(* Logix 5000 AddOnInstructionDefinition export AKD_Drive; software revision 19.01 *)

TYPE AKD_Status :   // All connections to the drive ethernet module are established and data is successfully transferring.
STRUCT
   Profile_In_Progress : BOOL;   // Profile Move In Progress
   Block_In_Execution : BOOL;   // Block In Execution
   On_Target_Position : BOOL;   // On Target Position (1=Current Position Equals Last Target Position)
   General_Fault : BOOL;   // General Fault
   Current_Direction : BOOL;   // Current Motor Direction (0=Reverse, 1=Forward)
   Home_Level : BOOL;   // Level of Home Input
   Reg_Level : BOOL;   // Level of Registration Input
   Enable : BOOL;   // State of Enable Output
   Fault_Input_Fault : BOOL;   // Fault Input Active
   Fwd_Limit : BOOL;   // Forward Input Active
   Rev_Limit : BOOL;   // Reverse Input Active
   Positive_Limit : BOOL;   // Positive Software Limit Exceeded
   Negative_Limit : BOOL;   // Negative Software Limit Exceeded
   FE_Fault : BOOL;   // Following Error Fault
   Block_Fault : BOOL;   // Block Execution Fault
   Load_Complete : BOOL;   // Command Message Successfully Loaded
END_STRUCT
END_TYPE

TYPE AKD_Axis :   // Axis Data:
STRUCT
   Control : AKD_Control;   // Control bits to send to the drive
   Status : AKD_Status;   // Status bits received from the drive
   Input : AB:ETHERNET_MODULE_SINT_64Bytes:I:0;   // Data from the drive
   Output : AB:ETHERNET_MODULE_SINT_64Bytes:O:0;   // Data to the drive
   ResponseMsgType : SINT;   // Response type contained in latest IO response from drive. Used to check for errors
   CommandTimeout : INT;   // Time to allow for command response from drive. Dependent on scan rate and communicaiton rate
   PositionFeedback : DINT;   // Actual Position Value
   VelocityFeedback : DINT;   // Actual Velocity Value
END_STRUCT
END_TYPE

TYPE AKD_Control :   // Send Explicit Message
STRUCT
   Load_Data_Start_Profile : BOOL;   // Load Command Data / Start Profile Move
   Start_Block : BOOL;   // Execute Command block or block chain
   Incremental : BOOL;   // Incremental Position (0=Absolute, 1=Incremental)
   Direction : BOOL;   // Direction in Velocity Mode (0=Reverse, 1=Forward)
   Smooth_Stop : BOOL;   // Smooth / Controlled Stop w/ Deceleration
   Hard_Stop : BOOL;   // Hard / Immediate Stop
   Reg_Arm : BOOL;   // Arm the Registration Input
   Enable : BOOL;   // Enable Output
END_STRUCT
END_TYPE

ADD_ON_INSTRUCTION AKD_Drive   (* revision 2.0, ExecutePrescan *)
// Drive Communication
VAR_IN_OUT
   Axis_Input : AB:ETHERNET_MODULE_SINT_64Bytes:I:0; {required}
   Axis_Output : AB:ETHERNET_MODULE_SINT_64Bytes:O:0; {required}
   Axis_Internal : AKD_Axis; {required}
END_VAR
VAR
   Command_Bytes : SINT[8];
   Response_Bytes : SINT[8];
END_VAR

ROUTINE Logic   (* ladder *)
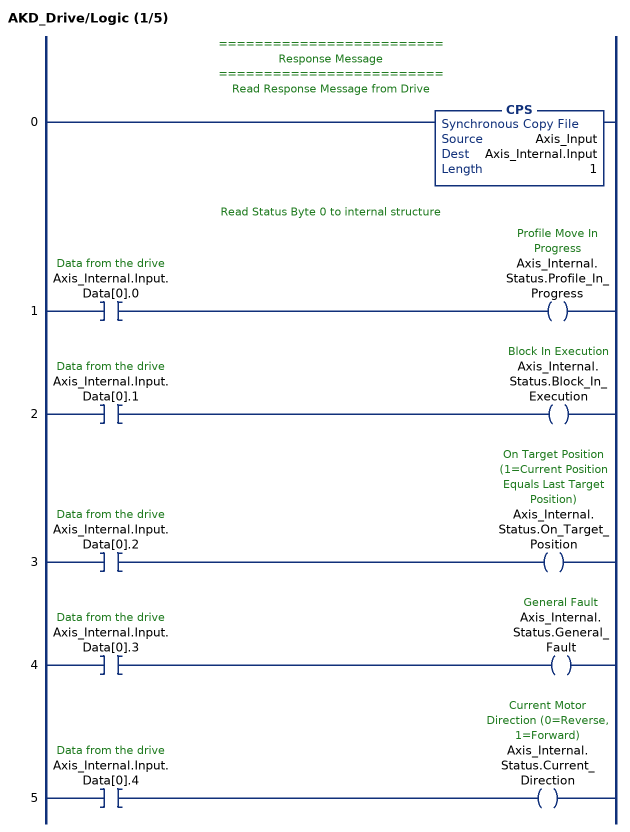
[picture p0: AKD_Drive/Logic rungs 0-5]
   // =========================
   // Response Message
   // =========================
   // Read Response Message from Drive
   0: CPS(Axis_Input,Axis_Internal.Input,1);
   // Read Status Byte 0 to internal structure
   1: XIC(Axis_Internal.Input.Data[0].0)OTE(Axis_Internal.Status.Profile_In_Progress);
   2: XIC(Axis_Internal.Input.Data[0].1)OTE(Axis_Internal.Status.Block_In_Execution);
   3: XIC(Axis_Internal.Input.Data[0].2)OTE(Axis_Internal.Status.On_Target_Position);
   4: XIC(Axis_Internal.Input.Data[0].3)OTE(Axis_Internal.Status.General_Fault);
   5: XIC(Axis_Internal.Input.Data[0].4)OTE(Axis_Internal.Status.Current_Direction);
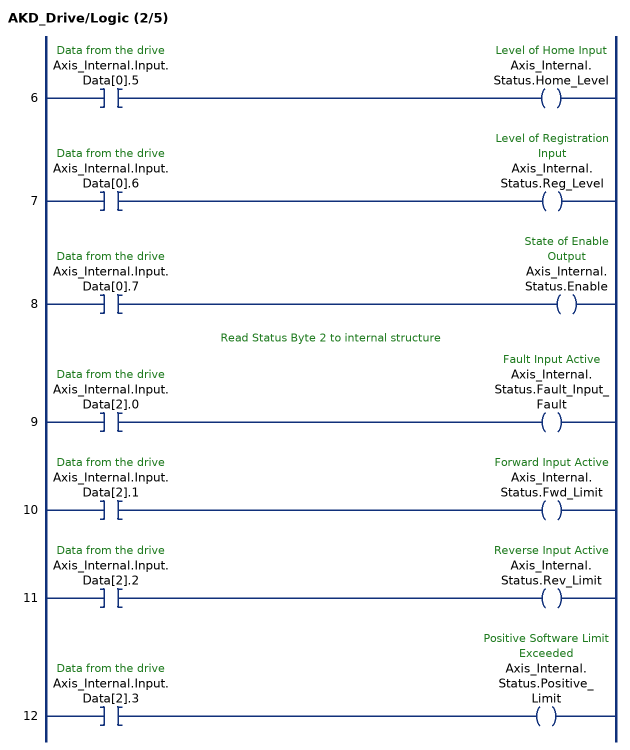
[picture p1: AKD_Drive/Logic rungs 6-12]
   6: XIC(Axis_Internal.Input.Data[0].5)OTE(Axis_Internal.Status.Home_Level);
   7: XIC(Axis_Internal.Input.Data[0].6)OTE(Axis_Internal.Status.Reg_Level);
   8: XIC(Axis_Internal.Input.Data[0].7)OTE(Axis_Internal.Status.Enable);
   // Read Status Byte 2 to internal structure
   9: XIC(Axis_Internal.Input.Data[2].0)OTE(Axis_Internal.Status.Fault_Input_Fault);
   10: XIC(Axis_Internal.Input.Data[2].1)OTE(Axis_Internal.Status.Fwd_Limit);
   11: XIC(Axis_Internal.Input.Data[2].2)OTE(Axis_Internal.Status.Rev_Limit);
   12: XIC(Axis_Internal.Input.Data[2].3)OTE(Axis_Internal.Status.Positive_Limit);
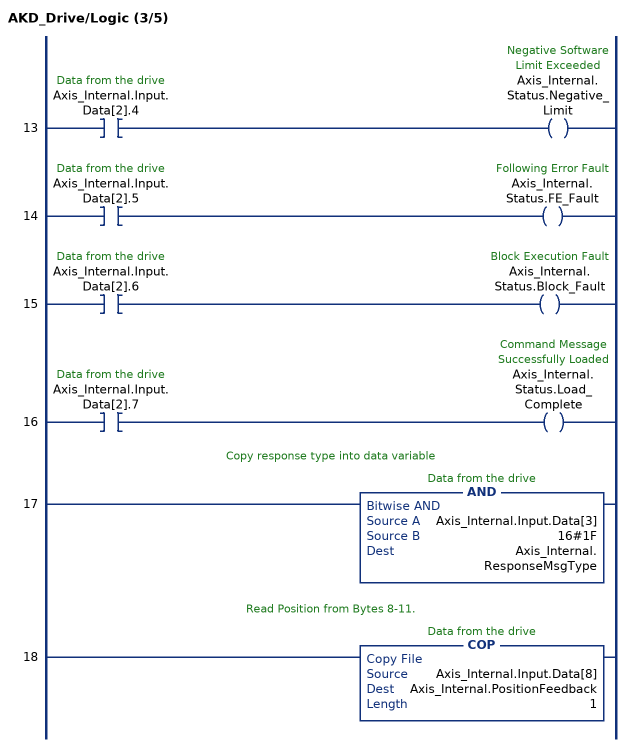
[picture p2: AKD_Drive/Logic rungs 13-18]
   13: XIC(Axis_Internal.Input.Data[2].4)OTE(Axis_Internal.Status.Negative_Limit);
   14: XIC(Axis_Internal.Input.Data[2].5)OTE(Axis_Internal.Status.FE_Fault);
   15: XIC(Axis_Internal.Input.Data[2].6)OTE(Axis_Internal.Status.Block_Fault);
   16: XIC(Axis_Internal.Input.Data[2].7)OTE(Axis_Internal.Status.Load_Complete);
   // Copy response type into data variable
   17: AND(Axis_Internal.Input.Data[3],16#1F,Axis_Internal.ResponseMsgType);
   // Read Position from Bytes 8-11.
   18: COP(Axis_Internal.Input.Data[8],Axis_Internal.PositionFeedback,1);
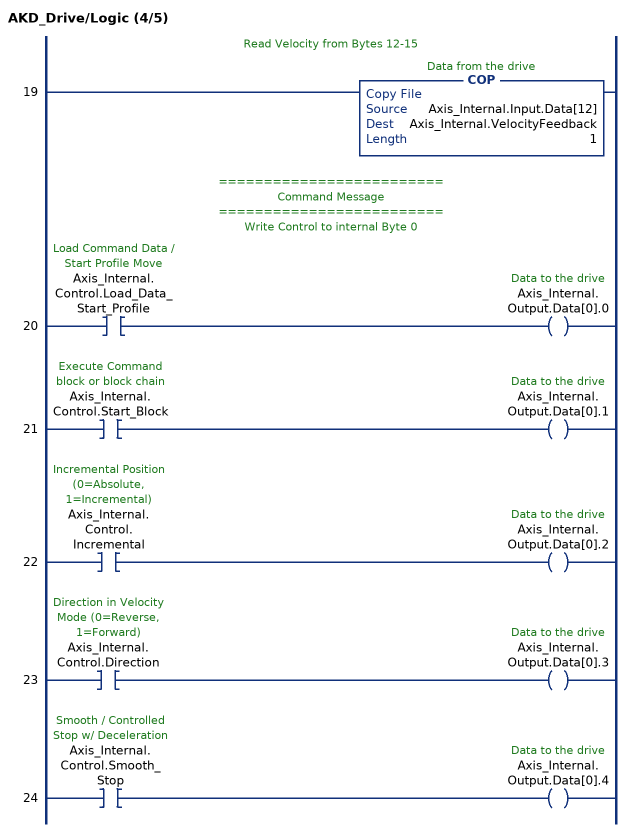
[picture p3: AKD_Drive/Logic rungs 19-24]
   // Read Velocity from Bytes 12-15
   19: COP(Axis_Internal.Input.Data[12],Axis_Internal.VelocityFeedback,1);
   // =========================
   // Command Message
   // =========================
   // Write Control to internal Byte 0
   20: XIC(Axis_Internal.Control.Load_Data_Start_Profile)OTE(Axis_Internal.Output.Data[0].0);
   21: XIC(Axis_Internal.Control.Start_Block)OTE(Axis_Internal.Output.Data[0].1);
   22: XIC(Axis_Internal.Control.Incremental)OTE(Axis_Internal.Output.Data[0].2);
   23: XIC(Axis_Internal.Control.Direction)OTE(Axis_Internal.Output.Data[0].3);
   24: XIC(Axis_Internal.Control.Smooth_Stop)OTE(Axis_Internal.Output.Data[0].4);
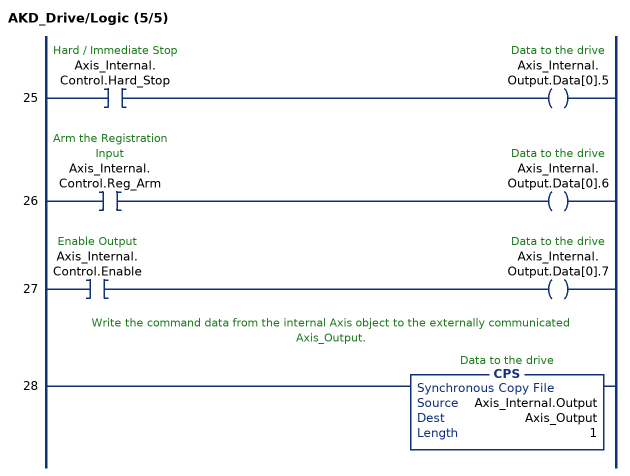
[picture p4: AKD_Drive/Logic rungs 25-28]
   25: XIC(Axis_Internal.Control.Hard_Stop)OTE(Axis_Internal.Output.Data[0].5);
   26: XIC(Axis_Internal.Control.Reg_Arm)OTE(Axis_Internal.Output.Data[0].6);
   27: XIC(Axis_Internal.Control.Enable)OTE(Axis_Internal.Output.Data[0].7);
   // Write the command data from the internal Axis object to the externally communicated Axis_Output.
   28: CPS(Axis_Internal.Output,Axis_Output,1);
END_ROUTINE

ROUTINE Prescan   (* ladder *)
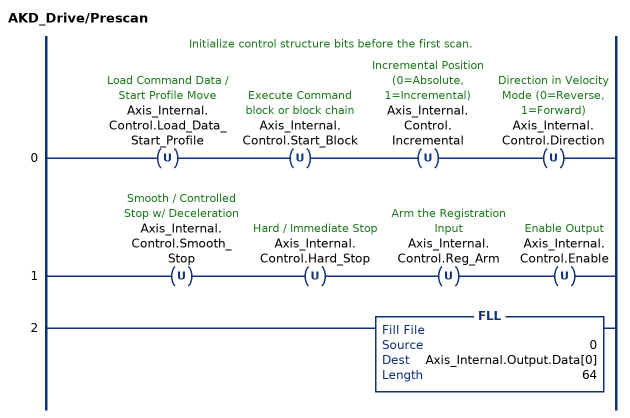
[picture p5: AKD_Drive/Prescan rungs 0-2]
   // Initialize control structure bits before the first scan.
   0: OTU(Axis_Internal.Control.Load_Data_Start_Profile)OTU(Axis_Internal.Control.Start_Block)OTU(Axis_Internal.Control.Incremental)OTU(Axis_Internal.Control.Direction);
   1: OTU(Axis_Internal.Control.Smooth_Stop)OTU(Axis_Internal.Control.Hard_Stop)OTU(Axis_Internal.Control.Reg_Arm)OTU(Axis_Internal.Control.Enable);
   2: FLL(0,Axis_Internal.Output.Data[0],64);
END_ROUTINE
END_ADD_ON_INSTRUCTION
